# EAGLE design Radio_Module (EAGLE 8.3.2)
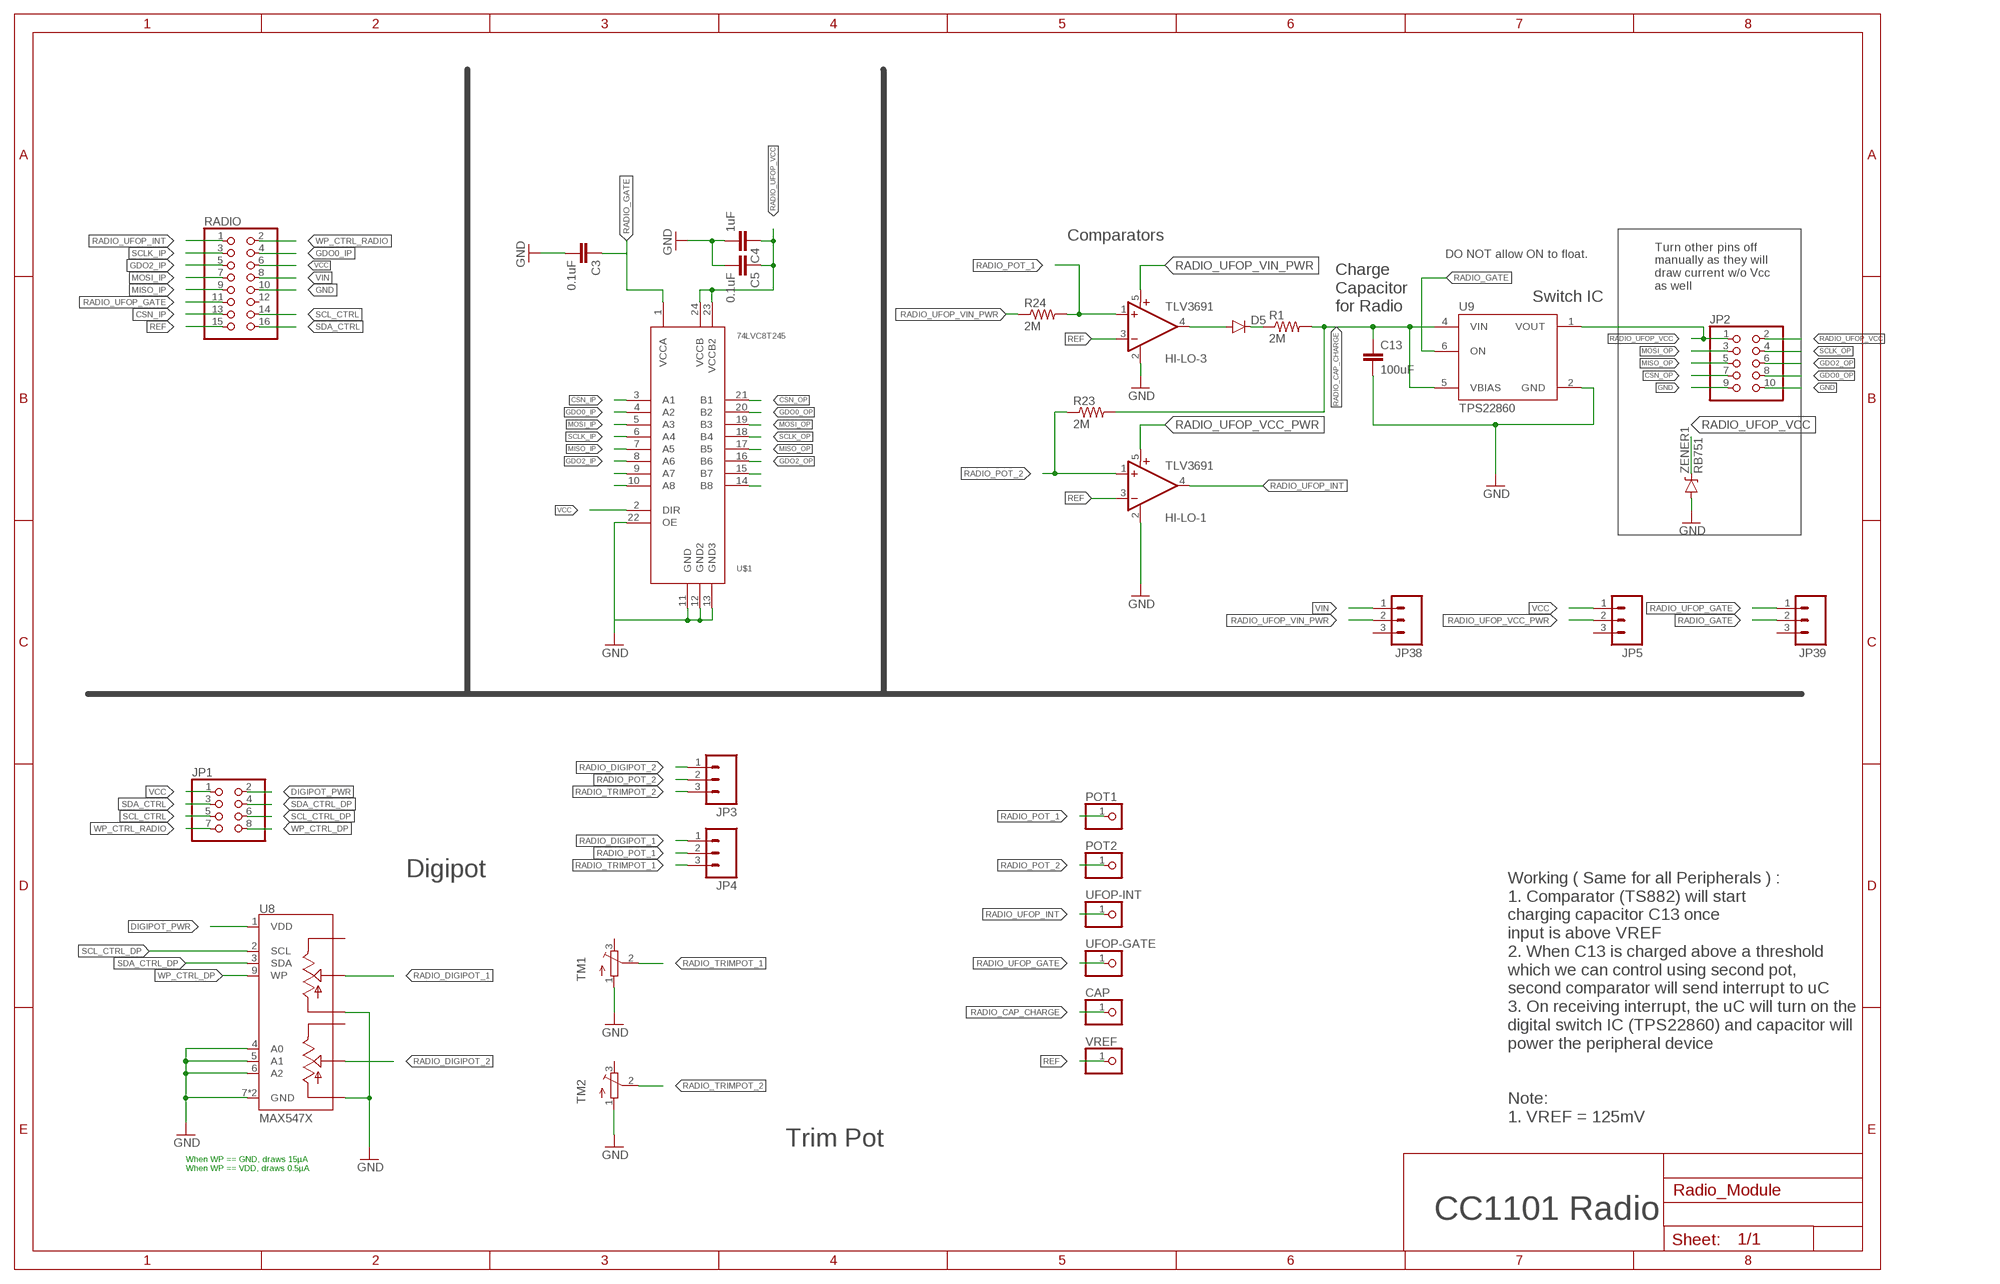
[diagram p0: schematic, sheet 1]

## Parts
C3  0.1uF  CAP0805  [0805]
C4  1uF  CAP0805  [0805]
C5  0.1uF  CAP0805  [0805]
C13  100uF  CAP0805  [0805]
CAP  PINHD-1X1  [1X01]
D5  DIODESOD523  [SOD523]
HI-LO-1  TLV3691  [SC70-5]
HI-LO-3  TLV3691  [SC70-5]
JP1  PINHD-2X4  [2X04]
JP2  PINHD-2X5  [2X05]
JP3  M03  [1X03-1.27MM]
JP4  M03  [1X03-1.27MM]
JP5  M03  [1X03-1.27MM]
JP38  M03  [1X03-1.27MM]
JP39  M03  [1X03-1.27MM]
POT1  PINHD-1X1  [1X01]
POT2  PINHD-1X1  [1X01]
R1  2M  RESISTOR0805-RES  [0805]
R23  2M  RESISTOR0805-RES  [0805]
R24  2M  RESISTOR0805-RES  [0805]
RADIO  PINHD-2X8/90  [2X08/90]
TM1  TRIMPOTTC33X  [TC33X]
TM2  TRIMPOTTC33X  [TC33X]
U8  MAX547X  [QFN16]
U9  TPS22860  [TSOT23-6]
U$1  74LVC8T245  [TSSOP24]
UFOP-GATE  PINHD-1X1  [1X01]
UFOP-INT  PINHD-1X1  [1X01]
VREF  PINHD-1X1  [1X01]
ZENER1  RB751  DIODE-ZENER  [SOD-523]

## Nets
CSN_IP: RADIO.13 U$1.3(A1)
CSN_OP: JP2.7 U$1.21(B1)
DIGIPOT_PWR: JP1.2 U8.1(VDD)
GDO0_IP: RADIO.4 U$1.4(A2)
GDO0_OP: JP2.8 U$1.20(B2)
GDO2_IP: RADIO.5 U$1.8(A6)
GDO2_OP: JP2.6 U$1.16(B6)
GND: C3.2 C4.2 C5.2 C13.2 HI-LO-1.2(GND) HI-LO-3.2(GND) JP2.9 JP2.10 RADIO.10 TM1.1(A) TM2.1(A) U8.4(A0) U8.5(A1) U8.6(A2) U8.7(GND) U8.10(LB) U8.13(LA) U8.TH(GND) U9.2(GND) U$1.11(GND) U$1.12(GND2) U$1.13(GND3) U$1.22(OE) ZENER1.ANODE(A)
MISO_IP: RADIO.9 U$1.7(A5)
MISO_OP: JP2.5 U$1.17(B5)
MOSI_IP: RADIO.7 U$1.5(A3)
MOSI_OP: JP2.3 U$1.19(B3)
N$1: D5.C R1.1
N$13: U$1.15(B7)
N$14: U$1.14(B8)
N$21: U$1.9(A7)
N$23: U$1.10(A8)
N$24: D5.A HI-LO-3.4(OUT)
RADIO_CAP_CHARGE: C13.1 CAP.1 R1.2 R23.2 U9.4(VIN) U9.5(VBIAS)
RADIO_DIGIPOT_1: JP4.1 U8.14(WA)
RADIO_DIGIPOT_2: JP3.1 U8.11(WB)
RADIO_GATE: C3.1 JP39.2 U9.6(ON) U$1.1(VCCA)
RADIO_POT_1: HI-LO-3.1(+IN) JP4.2 POT1.1 R24.2
RADIO_POT_2: HI-LO-1.1(+IN) JP3.2 POT2.1 R23.1
RADIO_TRIMPOT_1: JP4.3 TM1.2(S)
RADIO_TRIMPOT_2: JP3.3 TM2.2(S)
RADIO_UFOP_GATE: JP39.1 RADIO.11 UFOP-GATE.1
RADIO_UFOP_INT: HI-LO-1.4(OUT) RADIO.1 UFOP-INT.1
RADIO_UFOP_VCC: C4.1 C5.1 JP2.1 JP2.2 U9.1(VOUT) U$1.23(VCCB2) U$1.24(VCCB) ZENER1.CATHODE(C)
RADIO_UFOP_VCC_PWR: HI-LO-1.5(V+) JP5.2
RADIO_UFOP_VIN_PWR: HI-LO-3.5(V+) JP38.2 R24.1
REF: HI-LO-1.3(-IN) HI-LO-3.3(-IN) RADIO.15 VREF.1
SCL_CTRL: JP1.5 RADIO.14
SCL_CTRL_DP: JP1.6 U8.2(SCL)
SCLK_IP: RADIO.3 U$1.6(A4)
SCLK_OP: JP2.4 U$1.18(B4)
SDA_CTRL: JP1.3 RADIO.16
SDA_CTRL_DP: JP1.4 U8.3(SDA)
VCC: JP1.1 JP5.1 RADIO.6 U$1.2(DIR)
VIN: JP38.1 RADIO.8
WP_CTRL_DP: JP1.8 U8.9(WP)
WP_CTRL_RADIO: JP1.7 RADIO.2
Unconnected: JP5.3 JP38.3 JP39.3 RADIO.12 TM1.3(E) TM2.3(E) U8.12(HB) U8.15(HA)

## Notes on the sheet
- Comparators
- DO NOT allow ON to float.
- Charge 
  Capacitor 
  for Radio
- Turn other pins off 
  manually as they will
  draw current w/o Vcc
  as well
- Switch IC
- Digipot
- Working ( Same for all Peripherals ) :
  1. Comparator (TS882) will start 
  charging capacitor C13 once 
  input is above VREF
  2. When C13 is charged above a threshold
  which we can control using second pot, 
  second comparator will send interrupt to uC
  3. On receiving interrupt, the uC will turn on the
  digital switch IC (TPS22860) and capacitor will 
  power the peripheral device
- Note:
  1. VREF = 125mV
- Trim Pot
- When WP == GND, draws 15µA
  When WP == VDD, draws 0.5µA
- CC1101 Radio

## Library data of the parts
C3-C5 = SparkFun-Capacitors:CAP: Capacitor
C13 = SparkFun-Capacitors:CAP: Capacitor; DIGIKEY: 490-9969-1-ND
CAP POT1 POT2 UFOP-GATE UFOP-INT VREF = adafruit:PINHD-1X1: Pin header 1x1 for 0.1" spacing
D5 = SparkFun-DiscreteSemi:DIODE: Diode
HI-LO-1 HI-LO-3 = fedpower:TLV3691: 0.9-V to 6.5-V, Nanopower Comparator Datasheets Analog Signal Chain Guide TLV3691 Manufacturer Product Page TLV3691IDPFR Specifications Standard Package 1 CategoryIntegrated Circuits (ICs) FamilyLinear - Comparators Series- Packaging Cut Tape (CT) TypeGeneral Purpose Number of Elements1 Output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
JP1 = pinhead:PINHD-2X4: PIN HEADER
JP2 = pinhead:PINHD-2X5: PIN HEADER
JP3-JP5 JP38 JP39 = SparkFun-Connectors:M03: Header 3 Standard 3-pin 0.1" header. Use with straight break away headers (SKU : PRT-00116), right angle break away headers (PRT-00553), swiss pins (PRT-00743), machine pins (PRT-00117), and female headers (PRT-00115). Molex polarized connector foot print use with SKU : PRT-08232 with associated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
R1 R23 = SparkFun-Resistors:RESISTOR: Resistor; DIGIKEY: 311-2.00MHRCT-ND
R24 = SparkFun-Resistors:RESISTOR: Resistor
RADIO = pinhead:PINHD-2X8: PIN HEADER
TM1 TM2 = adafruit:TRIMPOT: SMT trimmer potentiometer part number TC33X http://www.ladyada.net/library/eagle
U8 = max547x:MAX547X: MAXIM MAX547X: Dual, 256-Tap, Nonvolatile, I2C-Interface, Digital Potentiometers, 400nA Iq, 250µA 12ms write The MAX5477/MAX5478/MAX5479 nonvolatile, dual, linear-taper, digital potentiometers perform the function of a mechanical potentiometer, but replace the mechanics with a simple 2-wire digital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; DIGIKEY: MAX5479ETE+-ND
U9 = tps22860:TPS22860: TI: TPS22860 Ultra-Low Leakage Load Switch The TPS22860 is a small, ultra-low leakage current, single channel load switch. The device requires a VBIAS voltage and can operate over an input voltage range of 0 V to VBIAS. It can support a maximum continuous current of 200 mA. The switch is controlled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; DIGIKEY: 296-43982-1-ND
U$1 = 74lvc8t245:74LVC8T245
ZENER1 = Parts:DIODE-ZENER: Zener Diode

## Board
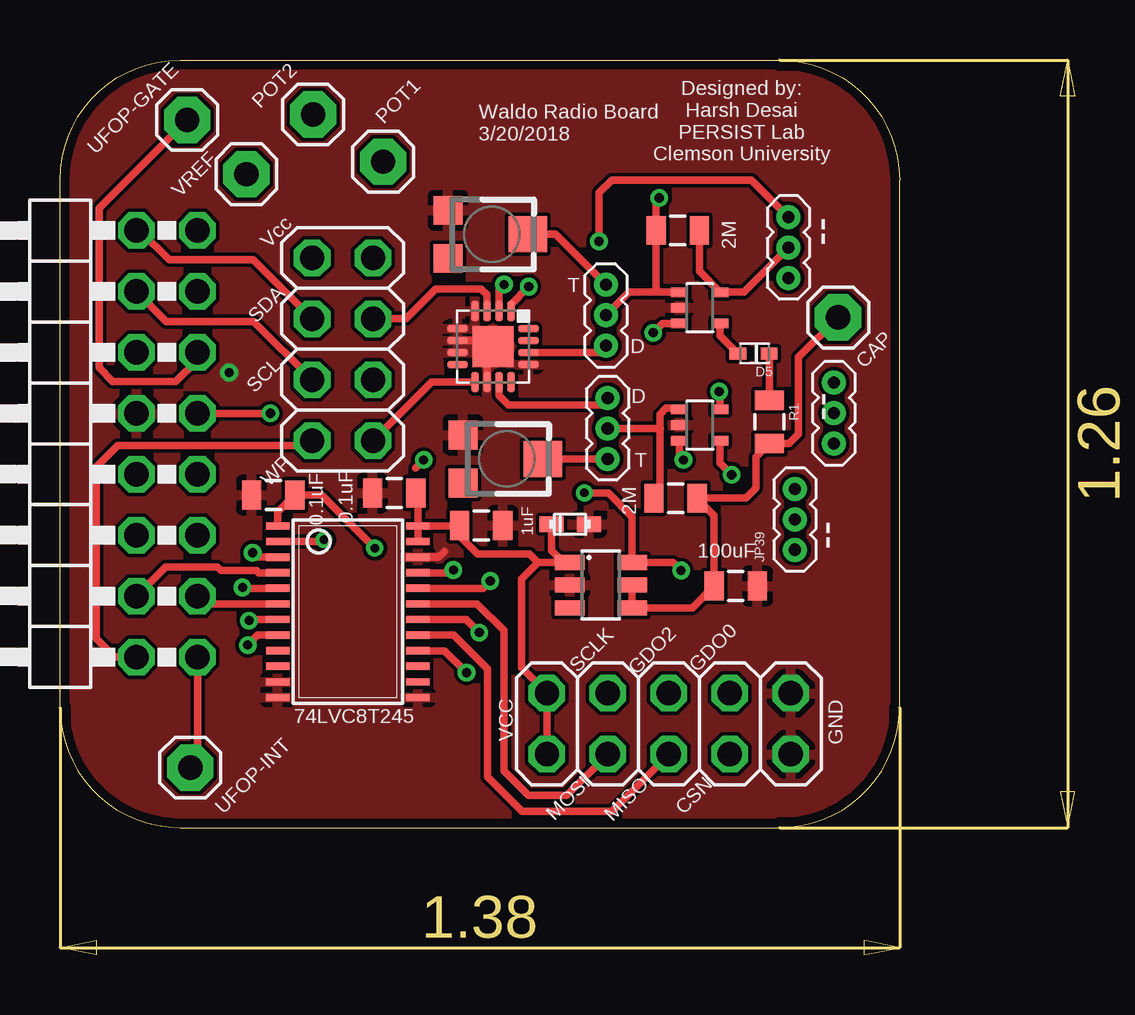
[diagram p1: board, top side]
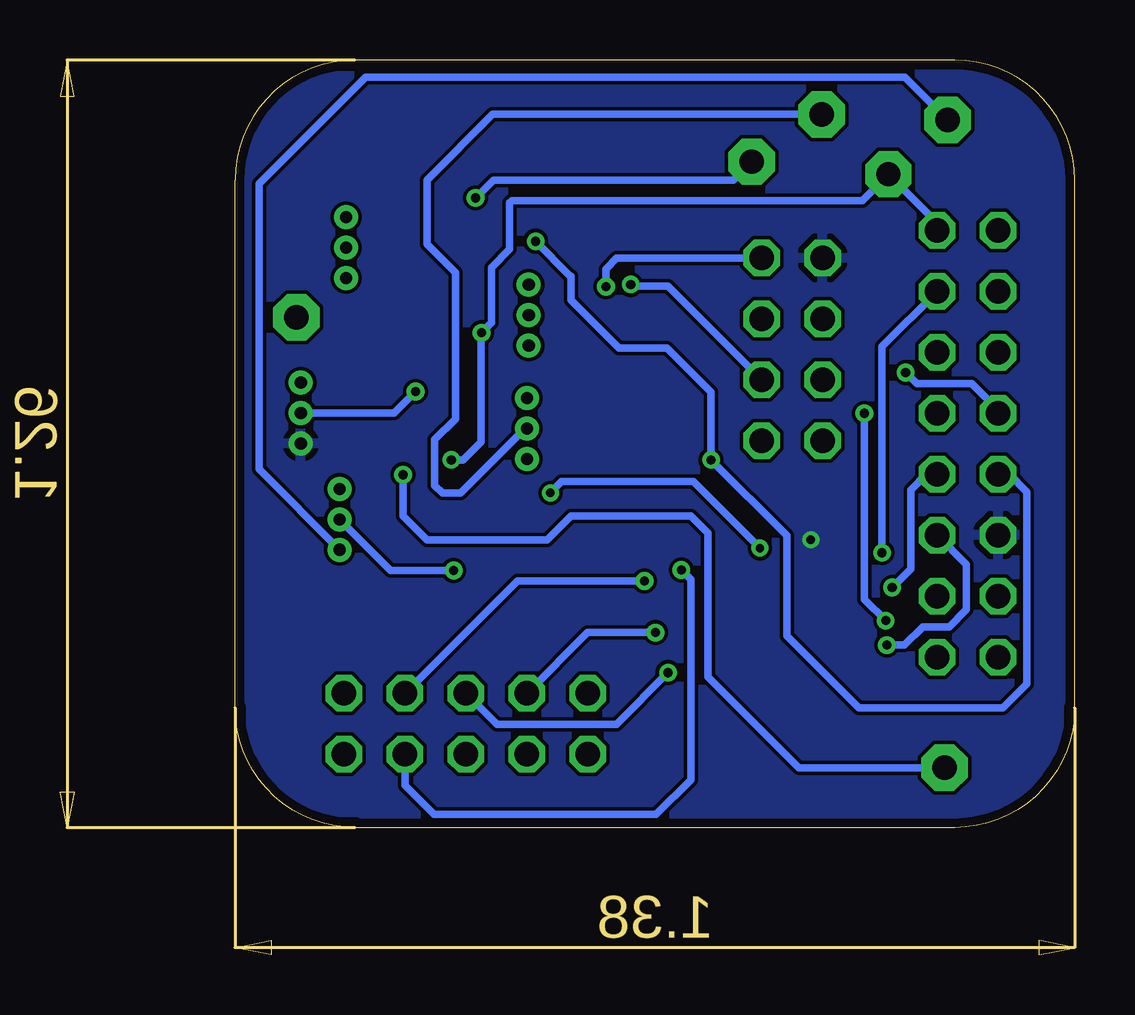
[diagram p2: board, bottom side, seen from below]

Size 42.3 x 37.3 mm. Coordinates in mm from the lower left corner, seen from the top.
Outline: 5,5.3 30,5.3 arc90 35,10.3 35,32.3 arc90 30,37.3 5,37.3 arc90 0,32.3 0,10.3 arc90 5,5.3
Copper layers (1*16): Top 0.0356mm / dielectric 1.5011mm / Bottom 0.0356mm
Design rules "oshpark-2layer": minimum track width 6mil, minimum drill 13mil, track to track 6mil, track to pad 6mil, pad to pad 6mil, via to via 6mil, smd to smd 6mil, copper to edge 15mil, drill to drill 6mil, minimum pad ring 7mil, minimum via ring 7mil, stop-mask expansion 2.5mil, vias tented up to drill 0mil, thermal gap 10mil

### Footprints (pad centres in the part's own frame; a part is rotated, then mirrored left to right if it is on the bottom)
0805 = smd 0.8 x 1.2: 1 -0.9,0; 2 0.9,0
1X01 = drill 1.016 pad 1.93 octagon: 1 0,0
SOD523 = smd 0.7 x 0.5: A 0.7,0; C -0.6,0
SC70-5 = smd 0.4 x 0.7: 1 -0.65,-0.85; 2 0,-0.85; 3 0.65,-0.85; 4 0.65,0.85; 5 -0.65,0.85
2X04 = drill 1.016 octagon: 1 -3.81,-1.27; 2 -3.81,1.27; 3 -1.27,-1.27; 4 -1.27,1.27; 5 1.27,-1.27; 6 1.27,1.27; 7 3.81,-1.27; 8 3.81,1.27
2X05 = drill 1.016 octagon: 1 -5.08,-1.27; 2 -5.08,1.27; 3 -2.54,-1.27; 4 -2.54,1.27; 5 0,-1.27; 6 0,1.27; 7 2.54,-1.27; 8 2.54,1.27; 9 5.08,-1.27; 10 5.08,1.27
1X03-1.27MM = drill 0.508 pad 1: 1 -1.27,0; 2 0,0; 3 1.27,0
2X08/90 = drill 1.016 octagon: 1 -8.89,-6.35; 2 -8.89,-3.81; 3 -6.35,-6.35; 4 -6.35,-3.81; 5 -3.81,-6.35; 6 -3.81,-3.81; 7 -1.27,-6.35; 8 -1.27,-3.81; 9 1.27,-6.35; 10 1.27,-3.81; 11 3.81,-6.35; 12 3.81,-3.81; 13 6.35,-6.35; 14 6.35,-3.81; 15 8.89,-6.35; 16 8.89,-3.81
TC33X = smd 1.2 x 1.2: 1 -1,-1.825; 3 1,-1.825 | smd 1.5 x 1.6: 2 0,1.5
QFN16 = smd 0.85 x 0.3: 1 -1.475,0.75; 2 -1.475,0.25; 3 -1.475,-0.25; 4 -1.475,-0.75; 9 1.475,-0.75; 10 1.475,-0.25; 11 1.475,0.25; 12 1.475,0.75 | smd 0.3 x 0.85: 5 -0.75,-1.475; 6 -0.25,-1.475; 7 0.25,-1.475; 8 0.75,-1.475; 13 0.75,1.475; 14 0.25,1.475; 15 -0.25,1.475; 16 -0.75,1.475 | smd 1.7 x 1.7: TH 0,0
TSOT23-6 = smd 0.62 x 1.22: 1 -0.95,-1.3; 2 0,-1.3; 3 0.95,-1.3; 4 0.95,1.3; 5 0,1.3; 6 -0.95,1.3
TSSOP24 = smd 0.305 x 0.991: 1 -3.575,-2.918; 2 -2.925,-2.918; 3 -2.275,-2.918; 4 -1.625,-2.918; 5 -0.975,-2.918; 6 -0.325,-2.918; 7 0.325,-2.918; 8 0.975,-2.918; 9 1.625,-2.918; 10 2.275,-2.918; 11 2.925,-2.918; 12 3.575,-2.918; 13 3.575,2.918; 14 2.925,2.918; 15 2.275,2.918; 16 1.625,2.918; 17 0.975,2.918; 18 0.325,2.918; 19 -0.325,2.918; 20 -0.975,2.918; 21 -1.625,2.918; 22 -2.275,2.918; 23 -2.925,2.918; 24 -3.575,2.918
SOD-523 = smd 1 x 0.635: ANODE -0.8,0; CATHODE 0.76,0

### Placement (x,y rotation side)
C3  8.89,19.16 180 top
C4  17.56,17.89 0 top
C5  13.93,19.25 180 top
C13  28.17,15.37 0 top
CAP  32.44,26.57 0 top
D5  28.96,25.07 180 top
HI-LO-1  26.67,22.08 270 top
HI-LO-3  26.67,26.97 270 top
JP1  11.78,25.24 270 top
JP2  25.38,9.63 0 top
JP3  22.83,21.94 270 top
JP4  22.76,26.66 90 top
JP5  32.26,22.58 90 top
JP38  30.37,29.48 270 top
JP39  30.64,18.15 90 top
POT1  13.47,33.06 0 top
POT2  10.55,35.03 0 top
R1  29.57,22.22 270 top
R23  25.66,19.03 0 top
R24  25.75,30.2 180 top
RADIO  -0.62,21.3 90 top
TM1  18,30.03 270 top
TM2  18.63,20.67 270 top
U8  18.05,25.35 270 top
U9  22.55,15.41 270 top
U$1  12,14.3 270 top
UFOP-GATE  5.3,34.8 0 top
UFOP-INT  5.43,7.8 0 top
VREF  7.77,32.54 0 top
ZENER1  21.26,17.94 180 top

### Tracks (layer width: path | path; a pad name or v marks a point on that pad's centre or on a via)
CSN_IP  (via drill 0.38)
  Top 0.305: U$1.3 8.22,16.57 v8.03,16.76
  Bottom 0.305: v8.03,16.76 8.03,25.35 RADIO.13
CSN_OP  (via drill 0.38)
  Top 0.305: U$1.21 16.29,15.93 v16.4,16.04
  Bottom 0.305: JP2.7 27.92,7.07 26.7,5.85 18,5.85 | 17.92,5.85 18,5.85 | 18,5.85 17.45,5.85 16,7.3 16,15.64 v16.4,16.04
DIGIPOT_PWR  (via drill 0.38)
  Top 0.305: U8.1 18.8,27.11 v19.54,27.85
  Bottom 0.305: v19.54,27.85 19.54,28.59 19.1,29.03 13.07,29.03 JP1.2
GDO0_IP
  Top 0.305: RADIO.4 4.4,16.16 6.56,16.16 6.71,16.01 8.2,16.01 8.29,15.93 U$1.4
GDO0_OP  (via drill 0.38)
  Top 0.305: v17.94,15.58 17.63,15.27 U$1.20
  Bottom 0.305: v17.94,15.58 23.24,15.58 JP2.8
GDO2_IP  (via drill 0.38)
  Top 0.305: U$1.8 8.24,13.32 v7.83,12.91
  Bottom 0.305: v7.83,12.91 7.1,12.91 6.34,13.67 5.23,13.67 4.51,14.39 4.51,16.27 RADIO.5
GDO2_OP  (via drill 0.38)
  Top 0.305: U$1.16 16.04,12.68 v16.95,11.76
  Bottom 0.305: v16.95,11.76 19.11,9.6 24.08,9.6 JP2.6
GND  (via drill 0.38)
  Top 0.305: U8.6 17.8,25.6 U8.TH 17.8,25.1 U8.10 | U$1.22 15.79,16.57 16.03,16.82
  Bottom 0.305: RADIO.10 3.19,22.7 4.3,23.81 6.59,23.81 v7.05,24.27
  pour Top: -1,38.3 -1,4.3 47,4.3 47,38.3
MISO_IP  (via drill 0.38)
  Top 0.305: U$1.7 7.92,13.98 v7.88,13.93 | v8.77,22.57 RADIO.9
  Bottom 0.305: v8.77,22.57 8.77,14.82 v7.88,13.93
MISO_OP
  Top 0.305: JP2.5 23,5.98 19.25,5.98 17.82,7.41 17.82,11.91 16.41,13.32 U$1.17
MOSI_IP  (via drill 0.38)
  Top 0.305: U$1.5 7.64,15.27 v7.61,15.31
  Bottom 0.305: RADIO.7 6.19,20.03 6.84,19.38 6.84,16.09 v7.61,15.32 v7.61,15.31
MOSI_OP
  Top 0.305: U$1.19 17.39,14.62 18.51,13.51 18.51,7.67 19.54,6.64 21.12,6.64 JP2.3
N$1
  Top 0.305: D5.C R1.1
N$24
  Top 0.305: HI-LO-3.4 27.52,25.81 D5.A
RADIO_CAP_CHARGE
  Top 0.305: R23.2 26.53,19 | 26.37,18.84 R23.2 | 29.01,20.7 29.01,20.3 | 29.01,20.3 29.01,19.45 28.59,19.03 R23.2 | 23.89,15.37 U9.5 U9.4 26.36,14.46 C13.1 27.27,18.32 R23.2 | 29.01,20.3 29.01,20.76 R1.2 30.39,21.32 30.79,21.71 30.79,24.92 CAP.1
RADIO_DIGIPOT_1
  Top 0.305: U8.14 22.47,25.1 JP4.1
RADIO_DIGIPOT_2
  Top 0.305: U8.11 18.3,23.31 18.69,22.92 22.54,22.92 JP3.1
RADIO_GATE  (via drill 0.35, 0.38)
  Top 0.305: v25.89,16.02 25.55,16.36 U9.6 23.85,18.26 22.86,19.25 v21.86,19.25 | U$1.1 9.08,18.46 C3.1 10.91,19.16 v13.12,16.95
  Bottom 0.305: v25.89,16.02 28.51,16.02 JP39.2 | v21.86,19.25 21.39,19.72 15.89,19.72 v13.12,16.95
RADIO_POT_1  (via drill 0.38)
  Top 0.305: 25,27.62 HI-LO-3.1 | 25,27.62 23.72,27.62 JP4.2 | 25,27.62 24.85,27.77 R24.2 24.85,31.42 v24.98,31.55
  Bottom 0.305: v24.98,31.55 24.23,32.3 14.23,32.3 POT1.1
RADIO_POT_2
  Top 0.305: JP3.2 25,21.94 | 25,21.94 25.03,21.94 | 25,21.94 25,22.52 25.27,22.79 25.76,22.79 HI-LO-1.1 | 25,21.94 25,19.27 R23.1
  Bottom 0.305: JP3.2 22.91,21.94 25.61,19.24 26.36,19.24 26.68,19.56 26.68,21.48 25.82,22.34 25.82,28.44 27,29.62 27,32.3 24.27,35.03 POT2.1
RADIO_TRIMPOT_1
  Top 0.305: TM1.2 20.66,30.03 JP4.3
RADIO_TRIMPOT_2
  Top 0.305: TM2.2 JP3.3
RADIO_UFOP_GATE
  Top 0.305: RADIO.11 5.73,24.8 4.83,23.9 2.2,23.9 1.63,24.47 1.63,31.13 UFOP-GATE.1
  Bottom 0.305: UFOP-GATE.1 7.09,36.59 29.55,36.59 34,32.14 34,20.24 JP39.1
RADIO_UFOP_INT  (via drill 0.38)
  Top 0.305: RADIO.1 5.73,8.1 UFOP-INT.1 | HI-LO-1.4 27.52,20.49 v28,20.01
  Bottom 0.305: UFOP-INT.1 11.5,7.8 15.29,11.59 15.29,17.58 16,18.29 16,18.3 21,18.3 22,17.3 27,17.3 28,18.3 v28,20.01
RADIO_UFOP_VCC
  Top 0.305: JP2.1 JP2.2 19.23,11.97 19.23,15.67 19.92,16.36 | 19.92,16.36 21,16.36 | 21,16.36 U9.1 | U$1.24 16.64,17.88 C4.1 16.66,17.45 17.41,16.7 19.58,16.7 19.92,16.36 | U$1.23 U$1.24 | U$1.24 14.92,19.16 C5.1 | ZENER1.CATHODE 20.5,16.86 21,16.36
RADIO_UFOP_VCC_PWR  (via drill 0.38)
  Top 0.305: HI-LO-1.5 27.52,23.44 v27.48,23.48
  Bottom 0.305: JP5.2 28.38,22.58 v27.48,23.48
RADIO_UFOP_VIN_PWR
  Top 0.305: R24.1 26.65,28.49 HI-LO-3.5 28.51,27.62 JP38.2
REF  (via drill 0.38)
  Top 0.305: HI-LO-3.3 25.12,26.32 v24.73,25.93 | HI-LO-1.3 25.82,20.8 v25.99,20.63
  Bottom 0.305: v25.99,20.63 25.49,20.63 24.74,21.38 v24.74,25.92 v24.73,25.93 24.31,26.35 24.31,28.65 23.55,29.41 23.55,31.35 23.46,31.44 8.86,31.44 VREF.1 | 5.73,30.46 RADIO.15 5.73,30.5 VREF.1 | VREF.1
SCL_CTRL
  Top 0.305: RADIO.14 4.43,26.4 8.08,26.4 JP1.5
SCL_CTRL_DP  (via drill 0.38)
  Top 0.305: v18.51,27.94 18.3,27.73 U8.2
  Bottom 0.305: JP1.6 16.95,27.87 18.44,27.87 v18.51,27.94
SCLK_IP
  Top 0.305: U$1.6 6.05,14.62 RADIO.3
SCLK_OP  (via drill 0.38)
  Top 0.305: U$1.18 16.93,13.98 v17.48,13.43
  Bottom 0.305: v17.48,13.43 20.31,13.43 JP2.4
SDA_CTRL
  Top 0.305: RADIO.16 3.33,30.19 4.55,28.97 8.05,28.97 JP1.3
SDA_CTRL_DP
  Top 0.305: JP1.4 14.42,26.51 15.66,27.75 17.56,27.75 17.8,27.51 U8.3
VCC  (via drill 0.35)
  Top 0.305: U$1.2 10.93,17.23 v11,17.3
  pour Bottom: -3,40.3 -3,2.3 49,2.3 49,40.3
VIN  (via drill 0.38)
  Top 0.305: 14.83,20.3 v15.16,20.63 | 22.47,30.17 v22.47,29.74 22.47,31.77 23,32.3 28.82,32.3 JP38.1
  Bottom 0.305: RADIO.8 2.73,20.03 2,19.3 2,11.3 3,10.3 9,10.3 12,13.3 12,17.47 v15.16,20.63 15.16,23.46 17,25.3 19,25.3 21,27.3 21,28.3 21.03,28.3 v22.47,29.74
WP_CTRL_DP
  Top 0.305: U8.9 15.49,23.88 JP1.8
WP_CTRL_RADIO
  Top 0.305: RADIO.2 2.29,12.41 1.51,13.19 1.51,20.34 2.4,21.23 10.31,21.23 JP1.7

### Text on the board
tPlace: Waldo Radio Board / 3/20/2018 | Designed by: / Harsh Desai / PERSIST Lab / Clemson University | -- | Vcc | T | SDA | D | SCL | D | -- | T | WP | -- | GDO0 | SCLK | GDO2 | VCC | GND | MOSI | MISO | CSN

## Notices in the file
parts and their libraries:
SparkFun-Capacitors: Licensing: Creative Commons ShareAlike 4.0 International - https://creativecommons.org/licenses/by-sa/4.0
